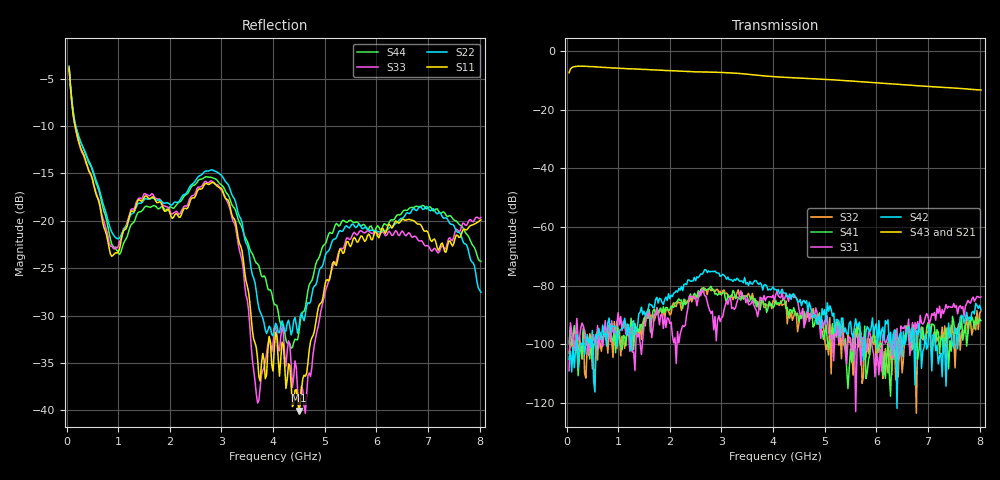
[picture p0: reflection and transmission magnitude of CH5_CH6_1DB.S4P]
!Agilent Technologies,E5071C,MY46316741,A.11.02
!Date: Mon Jun 01 10:40:00 2026
!Data & Calibration Information:
!1:CH5 INPUT 2:CH5 OUTPUT 3:CH6 INPUT 4:CH6 OUTPUT
!Freq	S11:SOLT4(ON)	S12:SOLT4(ON)	S13:SOLT4(ON)	S14:SOLT4(ON)
!	S21:SOLT4(ON)	S22:SOLT4(ON)	S23:SOLT4(ON)	S24:SOLT4(ON)
!	S31:SOLT4(ON)	S32:SOLT4(ON)	S33:SOLT4(ON)	S34:SOLT4(ON)
!	S41:SOLT4(ON)	S42:SOLT4(ON)	S43:SOLT4(ON)	S44:SOLT4(ON)
!PortZ  Port1:50+j0  Port2:50+j0  Port3:50+j0  Port4:50+j0
!Above PortZ is port z conversion or system Z0 setting when saving the data.
!When reading, reference impedance value at option line is always used.
# Hz S dB R 50
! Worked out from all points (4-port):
!   320 points, 50 MHz to 8.025 GHz, reference 50 ohm
!   strongest paths, dB at 50 MHz, 2.05 GHz, 4.05 GHz, 6.05 GHz, 8.025 GHz:
!     S43: -7.3, -6.7, -8.7, -10.9, -13.2
!     S21: -7.4, -6.9, -9.0, -11.1, -13.6
!     S42: -105.0, -83.7, -81.2, -91.9, -88.1
!     S31: -109.1, -96.9, -83.2, -110.4, -83.9
!     S41: -99.5, -87.2, -84.9, -100.7, -91.9
!     S32: -103.0, -86.7, -86.2, -102.8, -88.6
!   lowest |S11| = -40.0 dB at 4.5 GHz (marker M1), VSWR 1.02, Z = 49.5 - j0.88 ohm
!   |S11| at or under -10 dB: 165.5 MHz to end of sweep
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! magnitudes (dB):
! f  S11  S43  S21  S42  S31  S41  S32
! 50 MHz  -3.8  -7.3  -7.4  -105.0  -109.1  -99.5  -103.0
! 1.025 GHz  -23.0  -5.8  -6.0  -95.4  -93.3  -97.6  -95.4
! 3 GHz  -16.6  -7.3  -7.5  -76.5  -91.0  -82.8  -83.2
! 3.7 GHz  -34.6  -8.2  -8.4  -79.1  -90.6  -85.4  -87.1
! 4.5 GHz  -40.0  -9.2  -9.4  -85.6  -87.9  -92.3  -92.7
! 5.425 GHz  -22.2  -10.1  -10.3  -96.4  -106.7  -108.1  -103.2
! 8.025 GHz  -19.9  -13.2  -13.6  -88.1  -83.9  -91.9  -88.6
